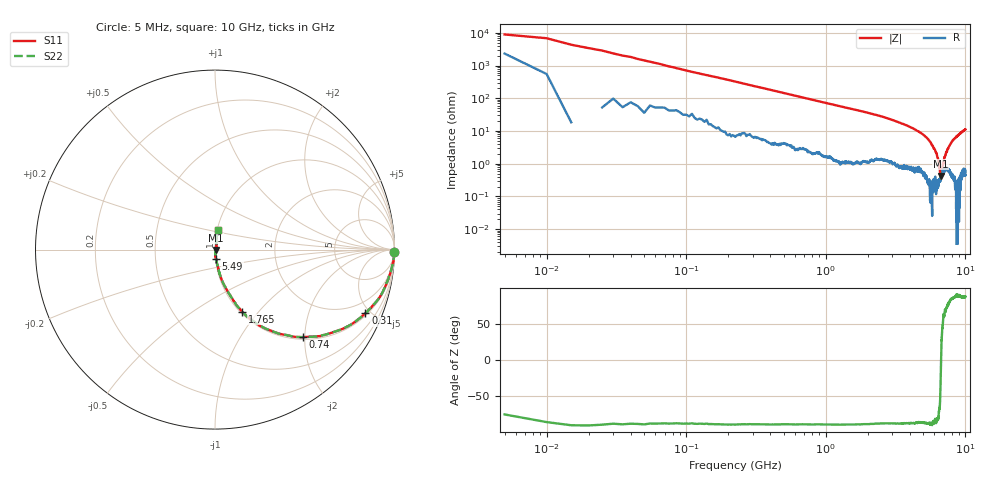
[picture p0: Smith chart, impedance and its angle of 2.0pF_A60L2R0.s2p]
! Amotech Co.,Ltd.
! http://www.amotech.co.kr/
! Part Number: A60L2R0
! These Parameters are Measured in Series Mode Connection
! Operation Temp=25[degC], DC Bias Voltage=0[V]
! Freq. Start=5[MHz] Stop=10[GHz], 2000[Steps]
! Date: Monday, July 14, 2020, 09:28:57
# GHZ S RI R 50.000000
!Freq.(Hz) S11(Real) S11(Imag) S21(Real) S21(Imag) S12(Real) S12(Imag) S22(Real) S22(Imag)
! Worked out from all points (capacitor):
!   2000 points, 5 MHz to 10 GHz, reference 50 ohm
!   read as one part in series: C = 2.24 pF near 55 MHz
!   lowest |Z| = 424 mohm at 6.635 GHz (marker M1)
!   series resonance near 6.692 GHz, so ESL is about 250 pH
!   S11 on the Smith chart (normalised r, x): 5 MHz: open; 310 MHz: 1.13, -4.67; 740 MHz: 1.05, -1.95; 1.765 GHz: 1.02, -0.82; 5.49 GHz: 1.01, -0.10; 10 GHz: 1.01, +0.23
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0.005  0.997 -0.0108  0.00305 0.0108  0.00305 0.0108  0.997 -0.0108
0.07  0.9857 -0.096  0.0143 0.096  0.0143 0.096  0.9857 -0.096
0.11  0.9687 -0.1498  0.0313 0.1498  0.0313 0.1498  0.9687 -0.1498
0.19  0.9308 -0.2416  0.0692 0.2416  0.0692 0.2416  0.9308 -0.2416
0.31  0.8384 -0.3542  0.1616 0.3542  0.1616 0.3542  0.8384 -0.3542
0.74  0.488 -0.4884  0.512 0.4884  0.512 0.4884  0.488 -0.4884
1.175  0.277 -0.438  0.723 0.438  0.723 0.438  0.277 -0.438
1.675  0.1636 -0.3571  0.8364 0.3571  0.8364 0.3571  0.1636 -0.3571
1.765  0.1505 -0.3452  0.8495 0.3452  0.8495 0.3452  0.1505 -0.3452
3.34  0.0391 -0.174  0.9609 0.174  0.9609 0.174  0.0391 -0.174
5.005  0.0102 -0.0748  0.9898 0.0748  0.9898 0.0748  0.0102 -0.0748
5.49  0.00542 -0.0504  0.9946 0.0504  0.9946 0.0504  0.00542 -0.0504
6.215  0.00281 -0.0205  0.9972 0.0205  0.9972 0.0205  0.00281 -0.0205
6.405  0.00238 -0.0128  0.9976 0.0128  0.9976 0.0128  0.00238 -0.0128
6.635  0.00347 -0.00241  0.9965 0.00241  0.9965 0.00241  0.00347 -0.00241
6.67  0.00426 -0.00121  0.9957 0.00121  0.9957 0.00121  0.00426 -0.00121
6.77  0.00421 0.00256  0.9958 -0.00256  0.9958 -0.00256  0.00421 0.00256
6.885  0.00664 0.00733  0.9934 -0.00733  0.9934 -0.00733  0.00664 0.00733
7.05  0.00738 0.0126  0.9926 -0.0126  0.9926 -0.0126  0.00738 0.0126
7.275  0.00746 0.0203  0.9925 -0.0203  0.9925 -0.0203  0.00746 0.0203
8.335  0.00672 0.0567  0.9933 -0.0567  0.9933 -0.0567  0.00672 0.0567
10  0.0169 0.1104  0.9831 -0.1104  0.9831 -0.1104  0.0169 0.1104
